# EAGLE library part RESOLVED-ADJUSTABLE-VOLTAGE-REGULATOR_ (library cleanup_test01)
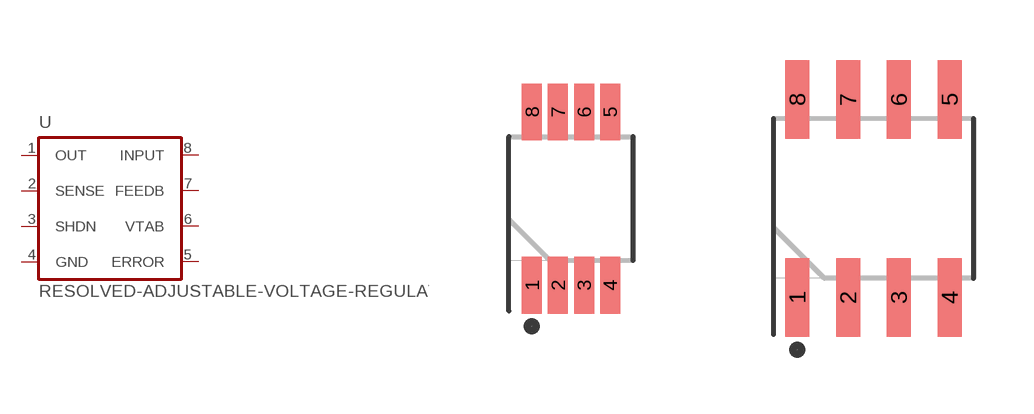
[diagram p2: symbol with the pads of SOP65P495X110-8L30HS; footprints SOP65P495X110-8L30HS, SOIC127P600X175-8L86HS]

Designator prefix -

## RESOLVED-ADJUSTABLE-VOLTAGE-REGULATOR_MSOP8  [SOP65P495X110-8L30HS]
1  OUT  out
2  SENSE  in
3  SHDN  in
4  GND  pwr
5  ERROR  out
6  VTAB  in
7  FEEDB  out
8  INPUT  pas

## RESOLVED-ADJUSTABLE-VOLTAGE-REGULATOR_SOIC8  [SOIC127P600X175-8L86HS]
Pads as for SOP65P495X110-8L30HS

## Footprint SOP65P495X110-8L30HS (pad centres in mm)
smd 0.5 x 1.42: 1 -0.975,-2.165; 2 -0.325,-2.165; 3 0.325,-2.165; 4 0.975,-2.165; 5 0.975,2.165; 6 0.325,2.165; 7 -0.325,2.165; 8 -0.975,2.165

## Footprint SOIC127P600X175-8L86HS (pad centres in mm)
smd 0.6 x 1.97: 1 -1.905,-2.475; 2 -0.635,-2.475; 3 0.635,-2.475; 4 1.905,-2.475; 5 1.905,2.475; 6 0.635,2.475; 7 -0.635,2.475; 8 -1.905,2.475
